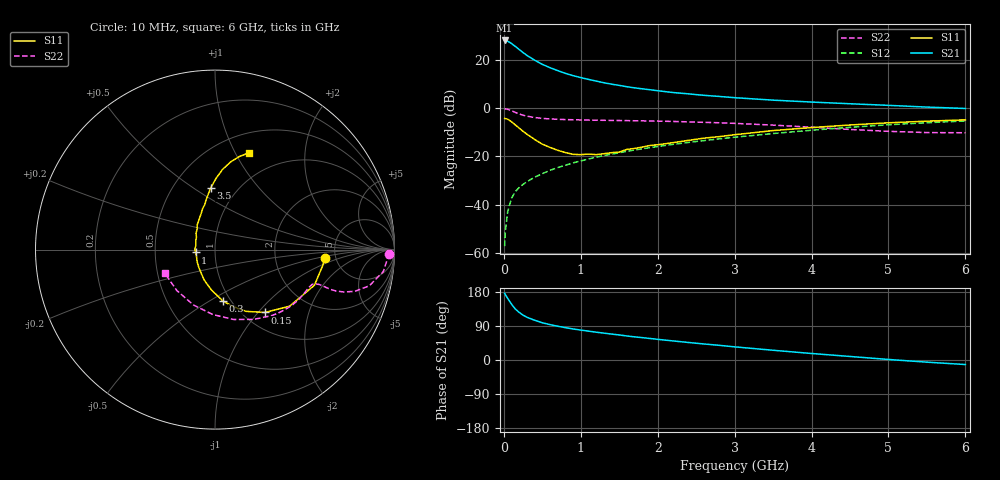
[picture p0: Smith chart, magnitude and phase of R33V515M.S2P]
! SIEMENS Small Signal Semiconductors
! BFR181
! Si NPN RF Bipolar Junction Transistor in SOT23
! VCE = 3.5 V  IC = 15 mA
! Common Emitter S-Parameters:  May  1996
# GHz  S  MA  R  50
!  f  S11  S21  S12  S22
! GHz  MAG  ANG  MAG  ANG  MAG  ANG  MAG  ANG
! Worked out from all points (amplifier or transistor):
!   36 points, 10 MHz to 6 GHz, reference 50 ohm
!   highest |S21| = 28.0 dB at 10 MHz (marker M1)
!   |S21| within 3 dB of that: start of sweep to 170 MHz
!   unconditionally stable (mu >= 1): 563.8 MHz to 2.58 GHz
!   at 250 MHz: K = 0.74, MSG = 27.2 dB, |S12| = -31.5 dB
!   at 1.4 GHz: K = 1.08, MAG = 12.7 dB, |S12| = -19.0 dB
!   at 6 GHz: K = 0.86, MSG = 2.6 dB, |S12| = -5.3 dB
!   S11 on the Smith chart (normalised r, x): 10 MHz: 4.07, -0.58; 150 MHz: 1.24, -1.09; 300 MHz: 0.92, -0.57; 1 GHz: 0.80, -0.03; 3.5 GHz: 0.76, +0.59; 6 GHz: 0.71, +1.14
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0.01  0.6121 -4.2  25.03 176.0  0.0014 84.7  0.9708 -1.3
0.02  0.6074 -8.2  24.87 172.4  0.0029 85.9  0.9625 -3.0
0.05  0.5885 -19.7  24.16 162.4  0.0072 81.2  0.9452 -7.5
0.1  0.5217 -37.2  21.66 147.3  0.0137 74.6  0.8831 -13.2
0.15  0.4474 -51.5  18.78 134.4  0.0189 71.6  0.8136 -16.6
0.2  0.3856 -63.2  16.24 125.5  0.0229 70.9  0.7563 -18.2
0.25  0.3315 -72.7  14.05 118.4  0.0265 69.0  0.7131 -18.9
0.3  0.2892 -81.3  12.31 112.8  0.0301 70.2  0.6811 -19.0
0.4  0.2253 -95.2  9.788 104.9  0.0373 69.9  0.6393 -18.7
0.5  0.1798 -109.6  8.03 98.2  0.0441 71.9  0.6136 -18.5
0.6  0.1542 -119.5  6.851 93.4  0.0517 72.4  0.5968 -18.7
0.7  0.1342 -132.2  5.96 89.1  0.0589 72.9  0.5872 -18.9
0.8  0.1206 -145.8  5.235 85.4  0.0659 72.7  0.5794 -19.3
1  0.109 -171.6  4.272 79.0  0.081 72.9  0.5704 -20.6
1.1  0.1122 178.4  3.922 76.2  0.0886 72.8  0.5656 -21.6
1.3  0.1139 159.2  3.345 70.9  0.1044 72.3  0.5592 -23.5
1.6  0.1402 139.0  2.769 63.4  0.128 71.0  0.5514 -27.1
2.2  0.1934 116.8  2.1 50.3  0.1781 67.6  0.5301 -35.6
3.5  0.3434 94.1  1.461 25.7  0.2982 56.4  0.4451 -60.8
4.5  0.4477 84.7  1.23 9.3  0.4009 44.9  0.362 -91.9
5.5  0.5371 75.2  1.05 -5.7  0.4988 31.3  0.3118 -133.0
6  0.5725 70.5  0.983 -12.0  0.5422 23.9  0.3095 -155.2
